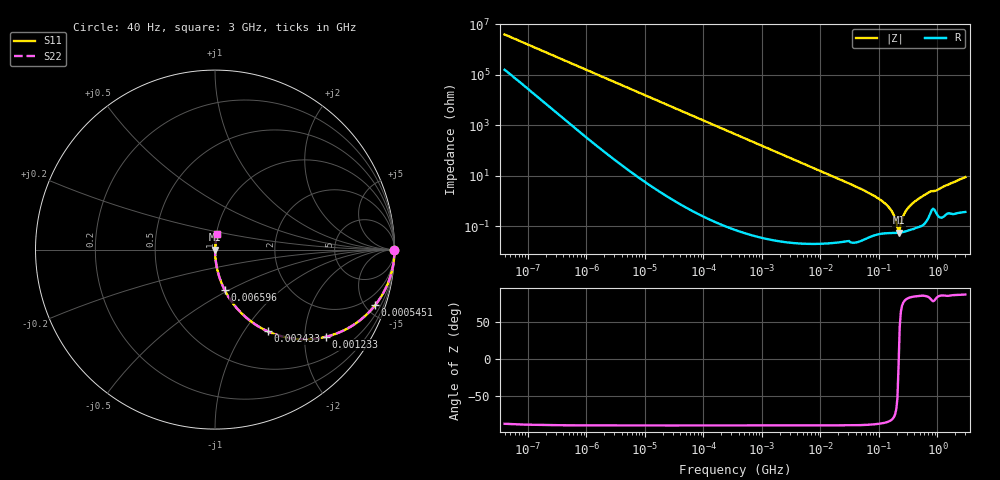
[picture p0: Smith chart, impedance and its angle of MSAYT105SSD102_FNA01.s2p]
! MSAYT105SSD102_FNA01  S-PARAMETER MODEL  ( General Type )
! Model Generated by TAIYO YUDEN Corporation (http://www.ty-top.com)
! Version 2.0
! TAIYO YUDEN Control No. 040624
! Copyright(c) 2004 TAIYO YUDEN CO.,LTD. All Rights Reserved.
! Product Description (link to TY-COMPAS)
! https://ds.yuden.co.jp/TYCOMPAS/or/detail?pn=MSAYT105SSD102KFNA01&u=M
! Products Name : Multilayer Ceramic Capacitors
! Characteristics :
!  Capacitance : 1000 pF , Rated Voltage : 25V
!  Case Size : 1.0 x 0.5 / 0.039 x 0.02 [mm/inch] , Thickness : 0.5 / 0.02 [mm/inch]
!  (Conditions: Temperature = 25 degC , DC Bias Current/Voltage = 0A / 0V)
! External Node Assignments :
!  1  o---| |---o  2
! GND o---------o GND
! Frequency Range : 40Hz  -  3GHz  [ 401 STEP ]
# MHz S RI R 50
! Freq[MHz].  S11 Real  S11 Imag  S21 Real  S21 Imag  S12 Real  S12 Imag  S22 Real  S22 Imag
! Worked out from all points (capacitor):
!   401 points, 40 Hz to 3 GHz, reference 50 ohm
!   read as one part in series: C = 1.02 nF near 44 Hz
!   lowest |Z| = 56.1 mohm at 216.4 MHz (marker M1)
!   series resonance near 217.7 MHz, so ESL is about 530 pH
!   S11 on the Smith chart (normalised r, x): 40 Hz: open; 545.1 kHz: 1.00, -5.74; 1.233 MHz: 1.00, -2.54; 2.433 MHz: 1.00, -1.29; 6.596 MHz: 1.00, -0.47; 3 GHz: 1.01, +0.18
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4e-05  1 -2.55e-05  1.02e-06 2.55e-05  1.02e-06 2.55e-05  1 -2.55e-05
0.000156  1 -9.96e-05  1.18e-06 9.96e-05  1.18e-06 9.96e-05  1 -9.96e-05
0.000834  1 -0.000533  1.59e-06 0.000533  1.59e-06 0.000533  1 -0.000533
0.017386  0.9999 -0.0111  0.000126 0.0111  0.000126 0.0111  0.9999 -0.0111
0.111532  0.9949 -0.0709  0.00506 0.0709  0.00506 0.0709  0.9949 -0.0709
0.362475  0.9491 -0.2197  0.0509 0.2197  0.0509 0.2197  0.9491 -0.2197
0.545089  0.8918 -0.3105  0.1082 0.3105  0.1082 0.3105  0.8918 -0.3105
1.232665  0.6172 -0.4859  0.3828 0.4859  0.3828 0.4859  0.6172 -0.4859
2.433099  0.2928 -0.4549  0.7072 0.4549  0.7072 0.4549  0.2928 -0.4549
6.596113  0.0534 -0.2244  0.9466 0.2244  0.9466 0.2244  0.0534 -0.2244
7.222098  0.045 -0.2068  0.955 0.2068  0.955 0.2068  0.045 -0.2068
66.58224  0.000807 -0.0212  0.9992 0.0212  0.9992 0.0212  0.000807 -0.0212
150.5692  0.000568 -0.00534  0.9994 0.00534  0.9994 0.00534  0.000568 -0.00534
172.504  0.000554 -0.00332  0.9994 0.00332  0.9994 0.00332  0.000554 -0.00332
206.7996  0.000551 -0.000726  0.9994 0.000726  0.9994 0.000726  0.000551 -0.000726
216.3901  0.000555 -8.48e-05  0.9994 8.48e-05  0.9994 8.48e-05  0.000555 -8.48e-05
236.926  0.00057 0.00119  0.9994 -0.00119  0.9994 -0.00119  0.00057 0.00119
259.4108  0.000601 0.00247  0.9994 -0.00247  0.9994 -0.00247  0.000601 0.00247
297.2015  0.000669 0.00445  0.9993 -0.00445  0.9993 -0.00445  0.000669 0.00445
427.1222  0.000969 0.0103  0.999 -0.0103  0.999 -0.0103  0.000969 0.0103
735.8749  0.0033 0.0227  0.9967 -0.0227  0.9967 -0.0227  0.0033 0.0227
3000  0.0115 0.0876  0.9885 -0.0876  0.9885 -0.0876  0.0115 0.0876
